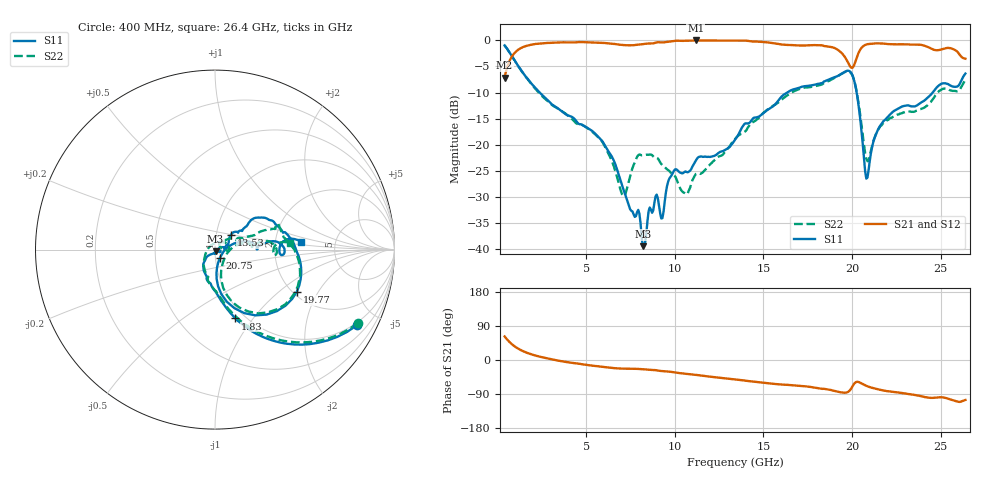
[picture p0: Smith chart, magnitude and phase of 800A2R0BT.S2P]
!  American Technical Ceramics  Date:  12/17/08
!  One Norden Lane
!  Huntington Station,  NY.  11746-2102
!  Tel:  (631) 622-4700  Fax:  (631) 622-4748
!  Part Number  800A2R0BT
!  Description: Broardband capacitor  Mounting Orientation: Vertical
!  Application:
# GHZ S DB R 50
! Freq  |S11|  S11 Ph  |S21|  S21 Ph  |S12|  S12 Ph  |S22|  S22 Ph
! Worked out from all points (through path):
!   401 points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, 400 MHz to 26.4 GHz, reference 50 ohm
!   highest |S21| = 0.00 dB at 11.19 GHz (marker M1); lowest = -7.2 dB at 400 MHz (marker M2)
!   group delay of S21, straight-line fit = 13.4 ps
!   lowest |S11| = -39.5 dB at 8.2 GHz (marker M3), VSWR 1.02, Z = 50.3 - j1.01 ohm
!   |S11| at or under -10 dB: 2.378 GHz to 16.34 GHz (13.96 GHz wide, 149 % of centre); 20.26 GHz to 24.55 GHz (4.292 GHz wide, 19.2 % of centre)
!   |S22| runs from -29.9 to -1.0 dB; largest |S21 - S12| = 0.005
!   S11 on the Smith chart (normalised r, x): 400 MHz: 0.89, -3.82; 1.83 GHz: 0.90, -0.82; 13.53 GHz: 1.18, +0.19; 19.77 GHz: 2.09, -1.34; 20.75 GHz: 1.05, -0.10; 26.4 GHz: 2.80, +0.33
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0.4  -0.95 -28.0  -7.18 62.1  -7.19 62.2  -0.96 -27.2
1.115  -4.64 -58.7  -1.92 31.4  -1.93 31.5  -4.66 -57.2
1.83  -7.95 -73.4  -0.87 16.2  -0.88 16.3  -8.04 -72.2
4.755  -16.16 -107.6  -0.31 -11.1  -0.32 -11.0  -16.21 -105.7
5.99  -19.78 -129.2  -0.47 -18.4  -0.47 -18.2  -19.94 -129.6
7.095  -28.53 -132.8  -0.88 -22.8  -0.87 -22.6  -29.88 130.8
8.2  -39.52 -71.5  -0.71 -24.3  -0.70 -24.1  -22.06 9.0
9.11  -31.70 -29.6  -0.34 -28.3  -0.32 -28.2  -22.99 -5.3
9.305  -34.13 4.6  -0.38 -29.2  -0.36 -29.0  -23.95 -3.2
9.89  -25.47 12.0  -0.13 -31.8  -0.11 -31.6  -25.85 4.5
10.54  -25.28 8.2  -0.06 -35.9  -0.05 -35.8  -29.27 26.8
11.19  -23.07 20.7  0.00 -39.2  -0.01 -39.1  -25.66 52.0
13.4  -19.09 41.1  -0.02 -51.3  -0.01 -51.3  -18.94 33.0
13.53  -18.45 42.6  -0.03 -51.9  -0.01 -51.9  -18.44 30.1
17.755  -8.60 21.1  -0.89 -71.9  -0.87 -72.0  -8.89 20.1
19.055  -7.01 1.9  -1.51 -82.1  -1.49 -82.1  -7.09 0.1
19.77  -5.80 -27.4  -4.18 -84.5  -4.17 -84.5  -5.92 -27.9
20.225  -9.25 -71.5  -3.75 -58.3  -3.72 -58.4  -9.12 -67.2
20.745  -25.19 -61.4  -0.86 -66.7  -0.84 -66.8  -21.67 -56.7
22.11  -14.35 14.0  -0.71 -82.9  -0.70 -83.1  -15.02 11.2
25.425  -8.39 -4.3  -1.43 -102.0  -1.42 -102.2  -9.35 -4.8
26.4  -6.37 5.3  -3.51 -105.5  -3.50 -105.6  -7.59 5.3
